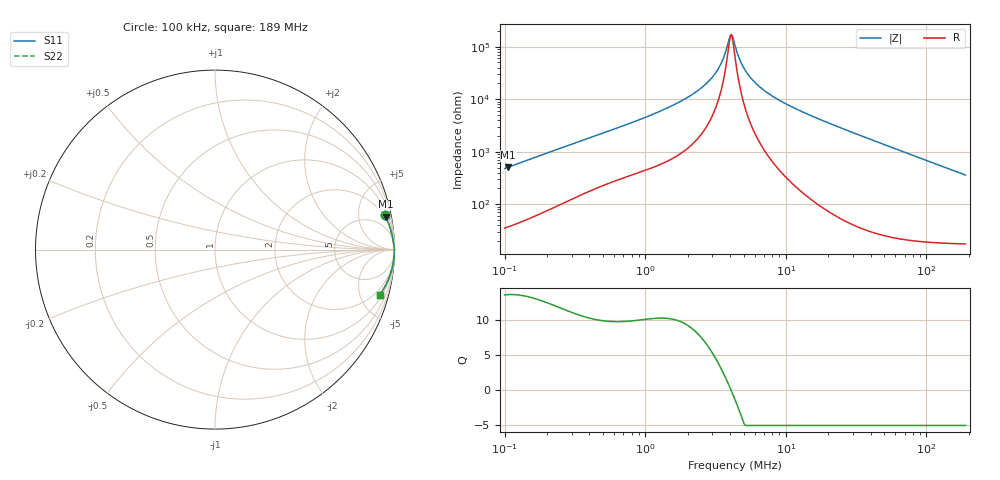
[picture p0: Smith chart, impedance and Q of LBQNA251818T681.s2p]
! LBQNA251818T681  S-PARAMETER MODEL  ( General Type )
! Model Generated by TAIYO YUDEN Corporation (http://www.ty-top.com)
! Version 1.0
! TAIYO YUDEN Control No. 191025NI43SB-FBB
! Copyright(c) 2019 TAIYO YUDEN CO.,LTD. All Rights Reserved.
! Product Description (link to TY-COMPAS)
! https://ds.yuden.co.jp/TYCOMPAS/or/detail?pn=LBQNA251818T681K&u=M
! Products Name : Inductors
! Characteristics :
!  Inductance : 680 uH , SRF(min) : 3.0 MHz , DC Resistance(max) : 22.1 Ohm
!  Rated Current : Saturation :30 mA , Temp Rise : 50 mA (20 degC)
!  Case Size : 2.5 x 1.8 / 0.098 x 0.071 [mm/inch] , Thickness : 1.8 / 0.071 [mm/inch]
!  (Conditions: Temperature = 25 degC , DC Bias Current/Voltage = 0A / 0V)
! External Node Assignments :
!  1  o---GGG---o  2
! GND o---------o GND
! Frequency Range : 0.1MHz  -  189.042664MHz  [ 402 STEP ]
# MHz S RI R 50
! Freq[MHz].  S11 Real  S11 Imag  S21 Real  S21 Imag  S12 Real  S12 Imag  S22 Real  S22 Imag
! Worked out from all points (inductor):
!   401 points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, 100 kHz to 189 MHz, reference 50 ohm
!   read as one part in series: L = 757 uH near 103.8 kHz
!   highest Q = 13.7 at 105.8 kHz (marker M1), where L = 761 uH
!   self-resonance near 4.032 MHz
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0.1  0.9454 0.1934  0.0546 -0.1934  0.0546 -0.1934  0.9454 0.1934
0.105822  0.9502 0.184  0.0498 -0.184  0.0498 -0.184  0.9502 0.184
0.353854  0.9906 0.0602  0.00938 -0.0602  0.00938 -0.0602  0.9906 0.0602
1.252125  0.998 0.0171  0.00196 -0.0171  0.00196 -0.0171  0.998 0.0171
1.93219  0.9989 0.00968  0.00112 -0.00968  0.00112 -0.00968  0.9989 0.00968
2.612836  0.9992 0.00549  0.000805 -0.00549  0.000805 -0.00549  0.9992 0.00549
2.981617  0.9993 0.00381  0.000715 -0.00381  0.000715 -0.00381  0.9993 0.00381
3.338876  0.9993 0.00242  0.000656 -0.00242  0.000656 -0.00242  0.9993 0.00242
3.600526  0.9994 0.00151  0.000624 -0.00151  0.000624 -0.00151  0.9994 0.00151
3.956607  0.9994 0.000382  0.000592 -0.000382  0.000592 -0.000382  0.9994 0.000382
4.031942  0.9994 0.000157  0.000586 -0.000157  0.000586 -0.000157  0.9994 0.000157
4.186944  0.9994 -0.000294  0.000576 0.000294  0.000576 0.000294  0.9994 -0.000294
4.347904  0.9994 -0.000745  0.000567 0.000745  0.000567 0.000745  0.9994 -0.000745
4.60102  0.9994 -0.00142  0.000556 0.00142  0.000556 0.00142  0.9994 -0.00142
4.961577  0.9995 -0.00234  0.000545 0.00234  0.000545 0.00234  0.9995 -0.00234
5.452262  0.9995 -0.0035  0.000536 0.0035  0.000536 0.0035  0.9995 -0.0035
6.221807  0.9995 -0.00519  0.000535 0.00519  0.000535 0.00519  0.9995 -0.00519
8.903343  0.9994 -0.0103  0.000595 0.0103  0.000595 0.0103  0.9994 -0.0103
15.38522  0.999 -0.021  0.000965 0.021  0.000965 0.021  0.999 -0.021
54.44117  0.9922 -0.0788  0.00778 0.0788  0.00778 0.0788  0.9922 -0.0788
101.448  0.9744 -0.1444  0.0256 0.1444  0.0256 0.1444  0.9744 -0.1444
189.0427  0.918 -0.251  0.082 0.251  0.082 0.251  0.918 -0.251
